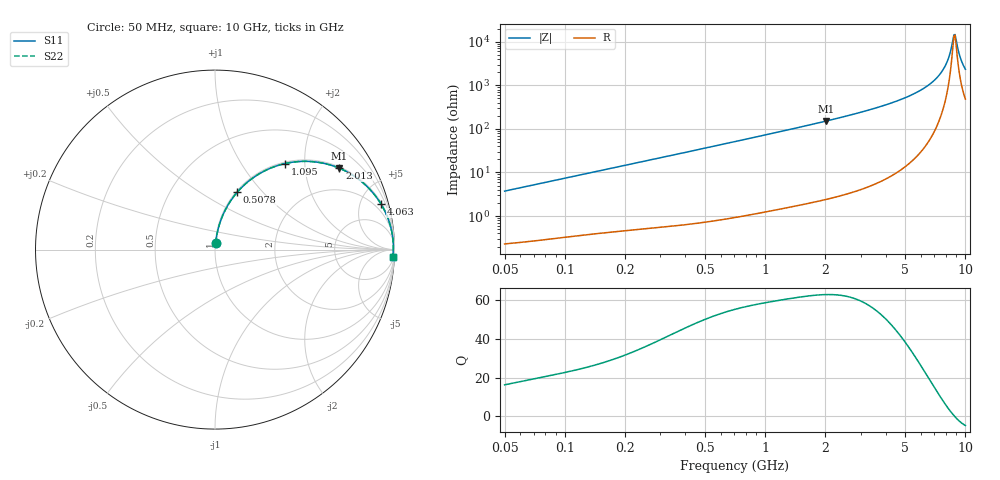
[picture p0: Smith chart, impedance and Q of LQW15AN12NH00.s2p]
!Murata Part Number: LQW15AN12NH00
!These Parameters are Measured in Series Mode Connection
!  o--[Z]--o
!Port1  Port2
!  o-------o
!Freq. Start=50[MHz] Stop=10[GHz], 401[Steps]
# Hz S RI R 50
!Freq.(Hz)	S 11(Real)	S 11(Imag)	S 21(Real)	S 21(Imag)	S 12(Real)	S 12(Imag)	S 22(Real)	S 22(Imag)
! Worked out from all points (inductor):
!   401 points, 50 MHz to 10 GHz, reference 50 ohm
!   read as one part in series: L = 11.8 nH near 51.34 MHz
!   highest Q = 62.8 at 2.013 GHz (marker M1), where L = 11.9 nH
!   self-resonance near 8.759 GHz
!   S11 on the Smith chart (normalised r, x): 50 MHz: 1.00, +0.07; 507.8 MHz: 1.01, +0.73; 1.095 GHz: 1.03, +1.59; 2.013 GHz: 1.05, +3.02; 4.063 GHz: 1.15, +7.28; 10 GHz: 11, -46
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5e7  0.00368 0.0371  0.9963 -0.0371  0.9963 -0.0371  0.00368 0.0371
1.214486e8  0.0114 0.0879  0.9886 -0.0879  0.9886 -0.0879  0.0114 0.0879
2.949953e8  0.0485 0.2023  0.9515 -0.2023  0.9515 -0.2023  0.0485 0.2023
5.077742e8  0.1236 0.3194  0.8764 -0.3194  0.8764 -0.3194  0.1236 0.3194
7.071068e8  0.2116 0.3995  0.7884 -0.3995  0.7884 -0.3995  0.2116 0.3995
1.094763e9  0.3897 0.4793  0.6103 -0.4793  0.6103 -0.4793  0.3897 0.4793
1.717543e9  0.6164 0.4783  0.3836 -0.4783  0.3836 -0.4783  0.6164 0.4783
2.013439e9  0.6928 0.4534  0.3072 -0.4534  0.3072 -0.4534  0.6928 0.4534
4.062795e9  0.9254 0.2528  0.0746 -0.2528  0.0746 -0.2528  0.9254 0.2528
4.171863e9  0.9306 0.2441  0.0694 -0.2441  0.0694 -0.2441  0.9306 0.2441
5.733131e9  0.9751 0.1397  0.0249 -0.1397  0.0249 -0.1397  0.9751 0.1397
7.086521e9  0.9897 0.0712  0.0103 -0.0712  0.0103 -0.0712  0.9897 0.0712
7.571744e9  0.9921 0.0499  0.00787 -0.0499  0.00787 -0.0499  0.9921 0.0499
7.983737e9  0.9933 0.0328  0.00672 -0.0328  0.00672 -0.0328  0.9933 0.0328
8.198065e9  0.9936 0.0242  0.00641 -0.0242  0.00641 -0.0242  0.9936 0.0242
8.644138e9  0.9937 0.00702  0.00633 -0.00702  0.00633 -0.00702  0.9937 0.00702
8.759398e9  0.9936 0.00269  0.00643 -0.00269  0.00643 -0.00269  0.9936 0.00269
8.876195e9  0.9934 -0.00164  0.00658 0.00164  0.00658 0.00164  0.9934 -0.00164
8.994549e9  0.9932 -0.00598  0.00678 0.00598  0.00678 0.00598  0.9932 -0.00598
9.48396e9  0.9919 -0.0234  0.00814 0.0234  0.00814 0.0234  0.9919 -0.0234
9.738562e9  0.9908 -0.0323  0.00919 0.0323  0.00919 0.0323  0.9908 -0.0323
1e10  0.9895 -0.0411  0.0105 0.0411  0.0105 0.0411  0.9895 -0.0411
